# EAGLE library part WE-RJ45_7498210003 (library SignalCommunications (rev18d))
WE-RJ45 LAN Transformer Order Code 7498210003 Design SMD xBase-T 10/100 Base-T Ports 1x1 Application Standard Tab Position UP LED (Left-Right) NO EMI Fingers No Details see: http://katalog.we-online.de/en/pbs/WE-LAN-RJ45 Created by Yingchun Shan 2016 (C) Wurth Elektronik
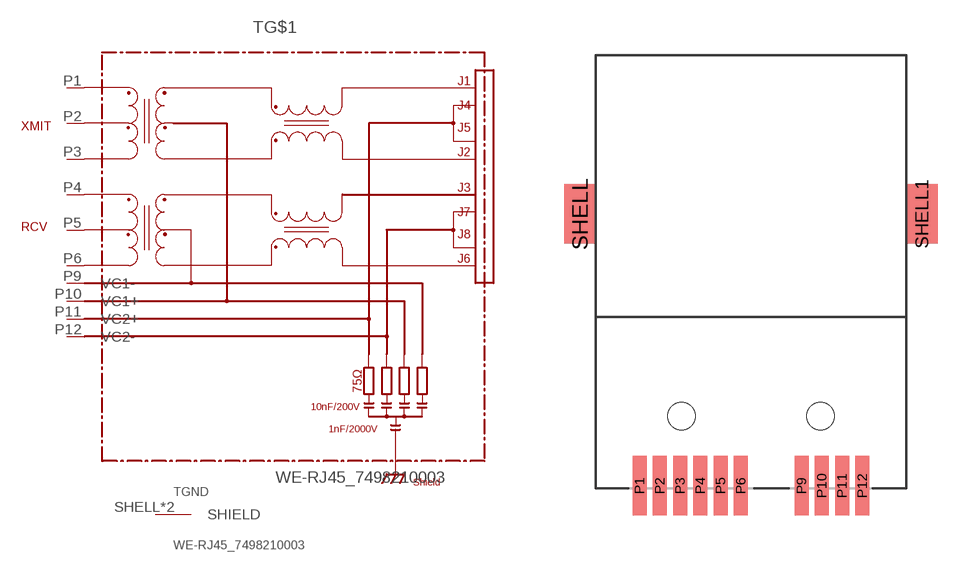
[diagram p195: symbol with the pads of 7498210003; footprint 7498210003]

Designator prefix T; gates G$1=7498210003 GND=SHIELD

## WE-RJ45_7498210003  [7498210003]
P1  G$1:P1
P2  G$1:P2
P3  G$1:P3
P4  G$1:P4
P5  G$1:P5
P6  G$1:P6
P9  G$1:VC1-
P10  G$1:VC1+
P11  G$1:VC2+
P12  G$1:VC2-
SHELL  GND:SHIELD  pas
SHELL1  GND:SHIELD  pas

## Footprint 7498210003 (pad centres in mm)
smd 0.71 x 3: P1 -5.61,-3.5; P2 -4.59,-3.5; P3 -3.57,-3.5; P4 -2.55,-3.5; P5 -1.53,-3.5; P6 -0.51,-3.5; P9 2.55,-3.5; P10 3.57,-3.5; P11 4.59,-3.5; P12 5.61,-3.5
smd 1.6 x 3: SHELL -8.61,10.2; SHELL1 8.61,10.2
hole 1.4 at -3.5,0
hole 1.4 at 3.5,0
